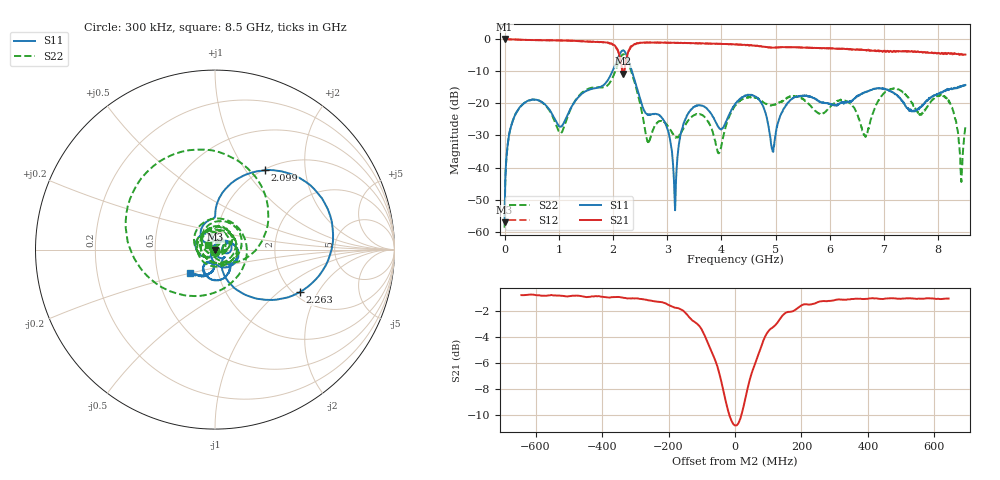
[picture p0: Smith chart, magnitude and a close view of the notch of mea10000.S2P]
!Agilent Technologies,E5071B,MY42402595,A.08.01
!Date: Tue Jan 02 09:02:02 2001
!Data & Calibration Information:
!Freq	S11:SOLT2(ON)	S21:SOLT2(ON)	S12:SOLT2(ON)	S22:SOLT2(ON)
# Hz S dB R 50
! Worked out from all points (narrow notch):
!   1601 points, 300 kHz to 8.5 GHz, reference 50 ohm
!   highest |S21| = 0.01 dB at 300 kHz (marker M1); lowest = -10.8 dB at 2.189 GHz (marker M2)
!   notch at M2: 8.8 dB deep, 107 MHz wide at half that depth
!   lowest |S11| = -57.0 dB at 300 kHz (marker M3), VSWR 1.00, Z = 50.1 - j0.111 ohm
!   |S11| at or under -10 dB: start of sweep to 1.989 GHz; 2.349 GHz to end of sweep
!   |S22| runs from -58.7 to -4.7 dB; largest |S21 - S12| = 0.035
!   S11 on the Smith chart (normalised r, x): 300 kHz: 1.00, -0.00; 2.099 GHz: 1.02, +1.24; 2.263 GHz: 2.17, -1.42; 8.5 GHz: 0.73, -0.20
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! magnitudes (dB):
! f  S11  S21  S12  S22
! 300 kHz  -57.0  0.0  -0.1  -58.7
! 79.98 MHz  -30.0  -0.1  -0.1  -30.1
! 260.6 MHz  -21.7  -0.2  -0.2  -21.7
! 1.036 GHz  -27.3  -0.4  -0.4  -29.3
! 1.419 GHz  -17.1  -0.7  -0.7  -16.8
! 2.099 GHz  -5.6  -4.0  -3.9  -7.4
! 2.189 GHz  -3.5  -10.8  -10.8  -4.7
! 2.263 GHz  -5.5  -5.1  -4.6  -6.5
! 2.635 GHz  -23.5  -1.1  -1.0  -31.9
! 2.837 GHz  -23.5  -1.1  -1.1  -25.7
! 3.145 GHz  -53.3  -1.2  -1.2  -30.4
! 3.416 GHz  -22.5  -1.3  -1.3  -24.7
! 3.953 GHz  -27.6  -1.4  -1.5  -35.6
! 4.25 GHz  -20.2  -1.7  -1.7  -20.8
! 4.691 GHz  -18.8  -2.2  -2.2  -18.6
! 4.946 GHz  -35.0  -2.7  -2.7  -20.5
! 5.669 GHz  -18.1  -2.7  -2.7  -21.2
! 6.651 GHz  -16.4  -3.4  -3.3  -30.1
! 7.087 GHz  -16.0  -4.0  -3.7  -15.9
! 8.149 GHz  -15.7  -4.6  -4.5  -18.4
! 8.42 GHz  -14.8  -4.8  -4.6  -43.7
! 8.5 GHz  -14.3  -4.8  -4.8  -27.3
